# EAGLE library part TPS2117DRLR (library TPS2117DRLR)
Power Switch ICs - Power Distribution 1.6-V to 5.5-V, 20-m?, 4-A low IQ power multiplexer with manual and priority switchover 8-SOT-5X3 -40 to 125 Source: Datasheet
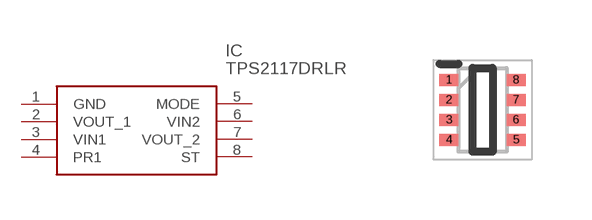
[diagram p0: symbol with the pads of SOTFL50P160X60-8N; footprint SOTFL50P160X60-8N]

Designator prefix IC

## TPS2117DRLR (Description: Power Switch ICs - Power Distribution 1.6-V to 5.5-V, 20-m?, 4-A low IQ power multiplexer with manual and priority switchover 8-SOT-5X3 -40 to 125; Height: 0.6mm; Manufacturer_Name: Texas Instruments; Manufacturer_Part_Number: TPS2117DRLR; Mouser_Part_Number: 595-TPS2117DRLR; Mouser_Price-Stock: https://www.mouser.co.uk/ProductDetail/Texas-Instruments/TPS2117DRLR?qs=HoCaDK9Nz5c%2FKe5lpCPPWQ%3D%3D)  [SOTFL50P160X60-8N]
1  GND
2  VOUT_1
3  VIN1
4  PR1
5  MODE
6  VIN2
7  VOUT_2
8  ST

## Footprint SOTFL50P160X60-8N (pad centres in mm)
DRL0008A
smd 0.475 x 0.3: 1 -0.838,0.75; 2 -0.838,0.25; 3 -0.838,-0.25; 4 -0.838,-0.75; 5 0.838,-0.75; 6 0.838,-0.25; 7 0.838,0.25; 8 0.838,0.75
